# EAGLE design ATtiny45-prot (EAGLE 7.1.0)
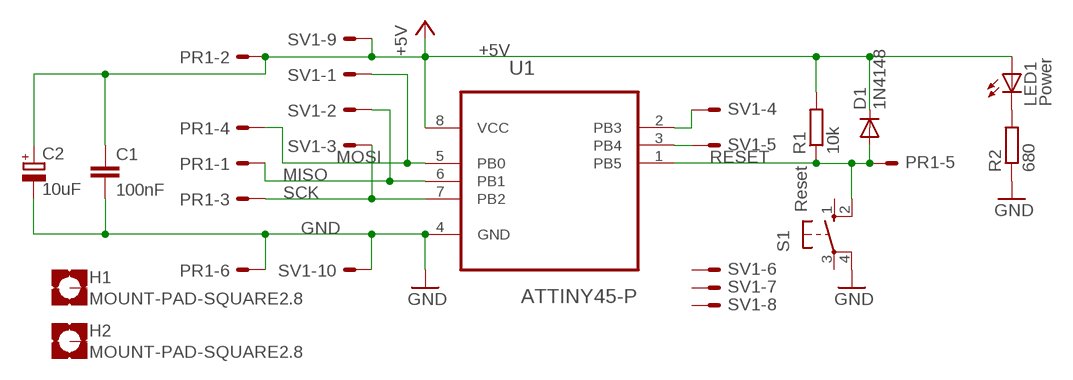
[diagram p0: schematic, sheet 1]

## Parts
C1  100nF  C-EU050-025W  [C050-025X075W]
C2  10uF  CPOL-EUE2.5-5  [E2,5-5]
D1  1N4148  [DO35]
H1  MOUNT-PAD-SQUARE2.8  [2,8-PAD-SQUARE]
H2  MOUNT-PAD-SQUARE2.8  [2,8-PAD-SQUARE]
LED1  Power  LED5MM  [LED5MM]
PR1  ML06E  [ML06]
R1  10k  R-EU_0207/10  [0207/10]
R2  680  R-EU_0207/10  [0207/10]
S1  Reset  40-XX  [TAST]
SV1  ML10EW  [ML10]
U1  ATTINY45-P  [DIP254P762X533-8]

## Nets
+5V: C1.1 C2.+ D1.C LED1.A PR1.2 R1.2 SV1.9 U1.8(VCC)
GND: C1.2 C2.- PR1.6 R2.1 S1.4(P1) SV1.10 U1.4(GND)
MISO: PR1.1 SV1.2 U1.6(PB1)
MOSI: PR1.4 SV1.1 U1.5(PB0)
N$6: SV1.5 U1.3(PB4)
N$7: SV1.4 U1.2(PB3)
N$8: LED1.K(C) R2.2
RESET: D1.A PR1.5 R1.1 S1.2(S1) U1.1(PB5)
SCK: PR1.3 SV1.3 U1.7(PB2)
Unconnected: H1.B2,8(MOUNT) H2.B2,8(MOUNT) S1.1(S) S1.3(P) SV1.6 SV1.7 SV1.8

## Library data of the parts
C1 = bar-rcl:C-EU: CAPACITOR, European symbol
C2 = bar-rcl:CPOL-EU: POLARIZED CAPACITOR, European symbol
D1 = bar-diode-trans:1N4148: DIODE
H1 H2 = holes:MOUNT-PAD-SQUARE: MOUNTING PAD, square
LED1 = bar-diode-trans:LED: LED
PR1 = bar-con:ML06E: ML06 6 pole flatcable connector used for Arduino programming ICSP
R1 R2 = bar-rcl:R-EU_: RESISTOR, European symbol
S1 = bar-switch:40-XX: OMRON SWITCH
SV1 = bar-con:ML10E: HARTING
U1 = bar-atmel:ATTINY45-P: 8-bit Microcontroller with 2/4/8KBytes In-System Programmable Flash; MPN: ATTINY45-20PU; OC_FARNELL: 1288352; OC_NEWARK: 23M5072; PACKAGE: PDIP-8; SUPPLIER: Atmel

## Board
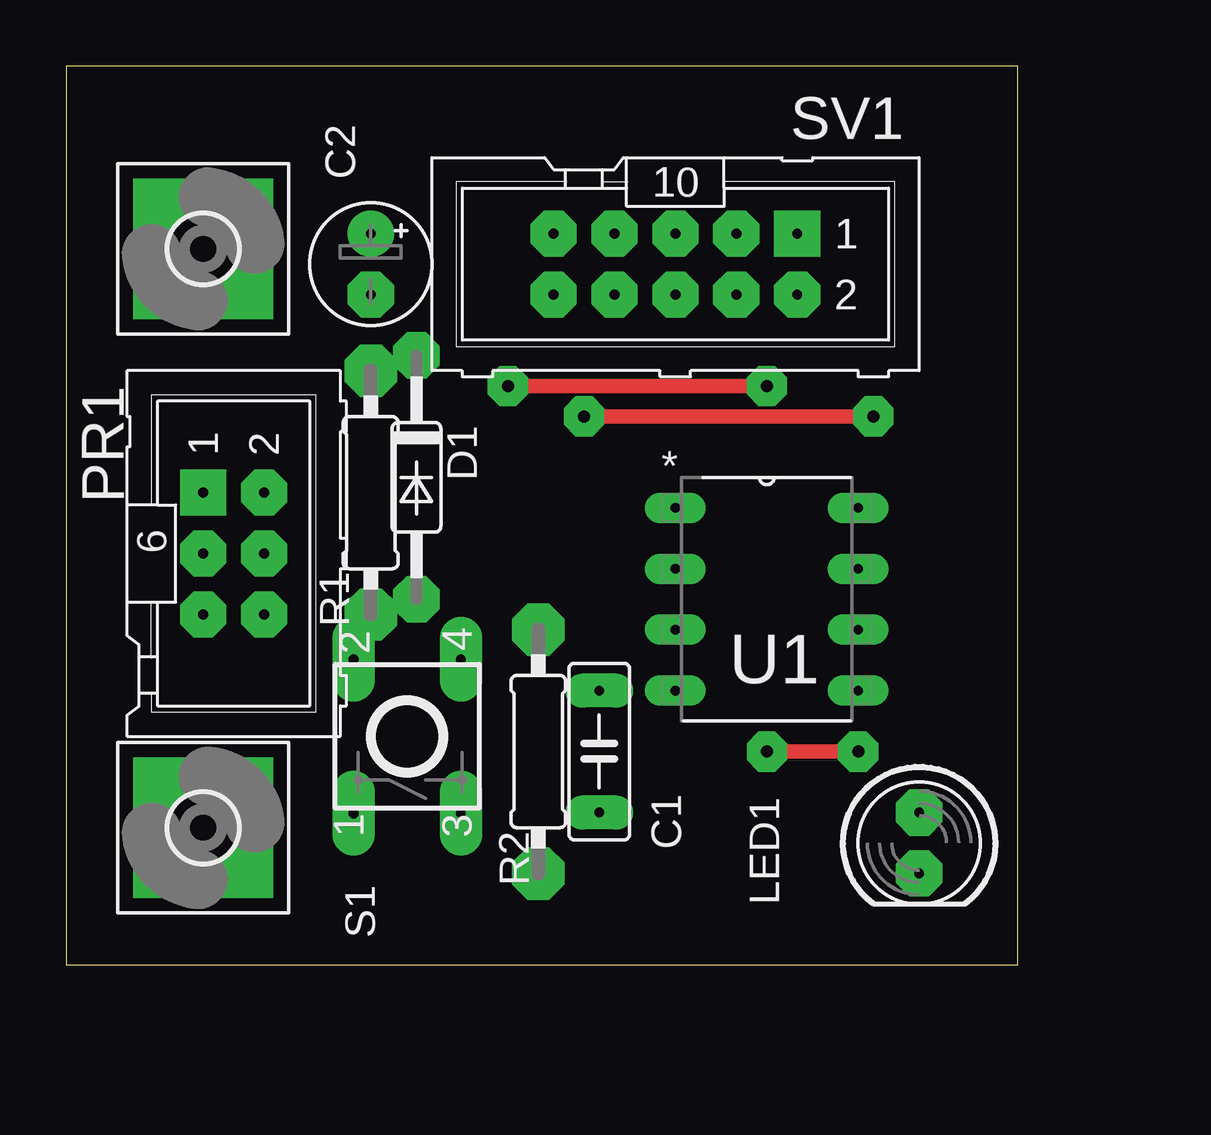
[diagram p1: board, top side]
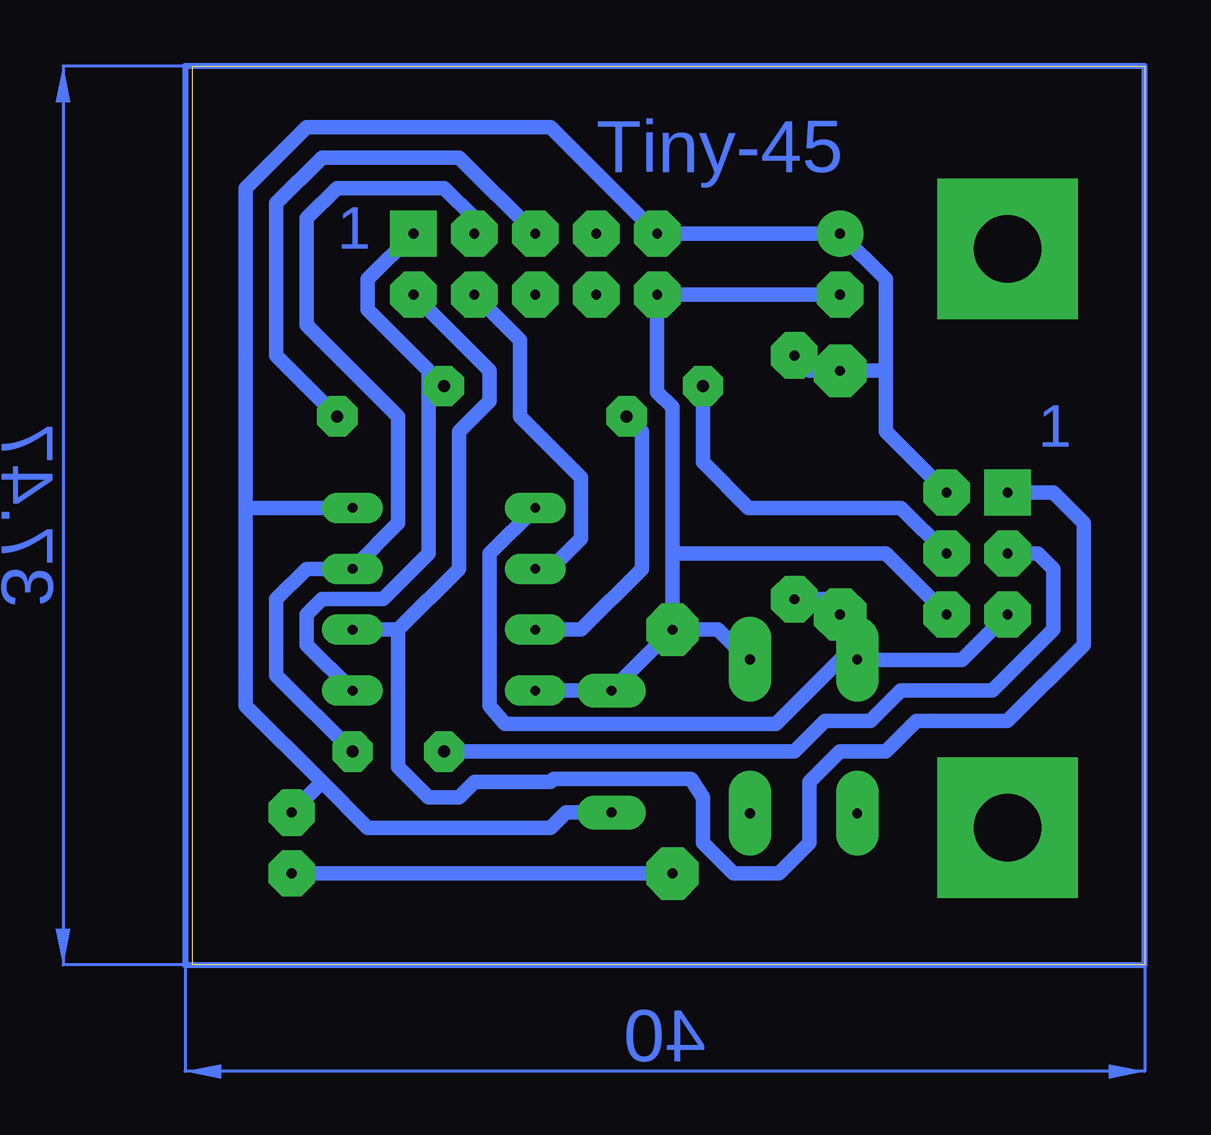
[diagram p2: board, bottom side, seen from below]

Size 39.67 x 37.45 mm. Coordinates in mm from the lower left corner, seen from the top.
Outline: 0,0 39.67,0 39.67,37.45 0,37.45 0,0
Copper layers (1*16): Top 0.035mm / dielectric 1.5mm / Bottom 0.035mm
Design rules "default": minimum track width 24mil, minimum drill 24mil, track to track 13mil, track to pad 13mil, pad to pad 13mil, via to via 13mil, smd to smd 13mil, copper to edge 40mil, drill to drill 8mil, minimum pad ring 10mil, minimum via ring 8mil, stop-mask expansion 4mil, vias tented up to drill 0mil, thermal gap 10mil

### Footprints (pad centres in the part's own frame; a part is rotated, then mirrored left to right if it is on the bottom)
C050-025X075W = drill 0.406 pad 1.422 long: 1 -2.54,0; 2 2.54,0
E2,5-5 = drill 0.406 pad 1.93: + -1.27,0 | drill 0.406 pad 1.93 octagon: - 1.27,0
DO35 = drill 0.406 pad 1.93 octagon: A 5.08,0; C -5.08,0
2,8-PAD-SQUARE = drill 2.8 pad 5.842 square: B2,8 0,0
LED5MM = drill 0.406 pad 1.93 octagon: A -1.27,0; K 1.27,0
ML06 = drill 0.406 pad 1.93 square: 1 -5.08,-1.27 | drill 0.406 pad 1.93 octagon: 2 -5.08,1.27; 3 -2.54,-1.27; 4 -2.54,1.27; 5 0,-1.27; 6 0,1.27
0207/10 = drill 0.406 pad 2.184 octagon: 1 -5.08,0; 2 5.08,0
TAST = drill 0.406 pad 1.778 long: 1 -3.208,1.989; 2 3.208,1.989; 3 -3.208,-2.489; 4 3.208,-2.489
ML10 = drill 0.406 pad 1.93 square: 1 -5.08,-1.27 | drill 0.406 pad 1.93 octagon: 2 -5.08,1.27; 3 -2.54,-1.27; 4 -2.54,1.27; 5 0,-1.27; 6 0,1.27; 7 2.54,-1.27; 8 2.54,1.27; 9 5.08,-1.27; 10 5.08,1.27
DIP254P762X533-8 = drill 0.406 pad 1.27 long: 1 -7.62,7.62; 2 -7.62,5.08; 3 -7.62,2.54; 4 -7.62,0; 5 0,0; 6 0,2.54; 7 0,5.08; 8 0,7.62

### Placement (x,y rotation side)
C1  22.22,8.89 90 top
C2  12.7,29.21 270 top
D1  14.6,20.32 270 top
H1  5.71,5.72 0 top
H2  5.71,29.84 0 top
LED1  35.56,5.08 270 top
PR1  6.98,14.61 270 top
R1  12.7,19.69 90 top
R2  19.68,8.89 270 top
S1  13.97,9.52 90 top
SV1  25.4,29.21 180 top
U1  33.02,11.43 0 top

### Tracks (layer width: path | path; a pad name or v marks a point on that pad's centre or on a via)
+5V
  Bottom 0.61: 10.79,24.77 R1.2 13.97,24.77 D1.C | 10.79,24.77 10.79,22.23 PR1.2 | 10.79,24.77 10.79,28.58 C2.+ SV1.9 24.76,34.92 34.92,34.92 37.47,32.38 37.47,19.05 | 34.29,7.62 32.39,5.72 24.76,5.72 24.13,6.35 C1.1 | 34.29,7.62 37.47,10.8 37.47,19.05 | U1.8 37.47,19.05 | LED1.A 34.29,7.62
GND
  Bottom 0.61: 19.68,17.15 10.79,17.15 PR1.6 | 19.68,17.15 19.68,23.24 20.32,23.88 SV1.10 C2.- | U1.4 C1.2 R2.1 | R2.1 19.68,17.15 | S1.4 16.54,12.73 17.78,13.97 R2.1
MISO
  Bottom 0.61: 31.11,13.97 U1.6 | 31.11,13.97 28.57,16.51 28.57,22.23 27.3,23.5 27.3,24.77 SV1.2 | 31.11,13.97 31.11,8.26 29.84,6.98 28.57,6.98 27.94,7.62 24.76,7.62 24.64,7.75 18.92,7.75 18.41,6.98 18.41,5.08 17.14,3.81 15.24,3.81 13.97,5.08 13.97,7.62 12.7,8.89 10.79,8.89 9.52,10.16 5.71,10.16 2.54,13.34 2.54,18.41 3.81,19.69 PR1.1
MOSI  (via drill 0.5 pad 1.68)
  Top 0.61: v18.41,24.13 v29.21,24.13
  Bottom 0.61: U1.5 34.92,13.34 34.92,14.61 34.29,15.24 31.75,15.24 29.84,17.15 29.84,24.13 | 29.84,24.13 29.84,24.77 32.39,27.3 32.39,28.58 SV1.1 | v18.41,24.13 18.41,20.95 16.51,19.05 10.16,19.05 PR1.4 | v29.21,24.13 29.84,24.13
N$5
  Bottom 0.254: 0,0 0,37.47 40,37.47 40,0 0,0
N$6  (via drill 0.5 pad 1.68)
  Top 0.61: v21.59,22.86 v33.66,22.86
  Bottom 0.61: U1.3 23.5,13.97 20.96,16.51 20.96,22.23 v21.59,22.86 | v33.66,22.86 36.19,25.4 36.19,31.75 34.29,33.66 28.57,33.66 SV1.5
N$7
  Bottom 0.61: U1.2 24.76,16.51 23.5,17.78 23.5,20.32 26.04,22.86 26.04,26.04 SV1.4
N$8
  Bottom 0.61: R2.2 LED1.K
RESET
  Bottom 0.61: D1.A 13.33,15.24 R1.1 11.98,13.89 S1.2 | PR1.5 7.62,12.7 11.95,12.7 S1.2 | U1.1 27.3,17.15 27.3,10.8 26.67,10.03 15.37,10.03 12.7,12.7 12.01,12.7 S1.2
SCK  (via drill 0.5 pad 1.68)
  Top 0.61: v29.21,8.89 v33.02,8.89
  Bottom 0.61: SV1.3 27.94,31.12 29.21,32.38 33.66,32.38 34.92,31.12 34.92,26.67 31.11,22.86 31.11,18.41 U1.7 34.92,16.51 36.19,15.24 36.19,12.06 v33.02,8.89 | v29.21,8.89 14.6,8.89 13.33,10.16 11.43,10.16 10.16,11.43 6.35,11.43 3.81,13.97 3.81,16.51 4.44,17.15 PR1.3
(copper drawn outside any net)
  shapes: Bottom area x2

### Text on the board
Bottom: Tiny-45 | 1 | 1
